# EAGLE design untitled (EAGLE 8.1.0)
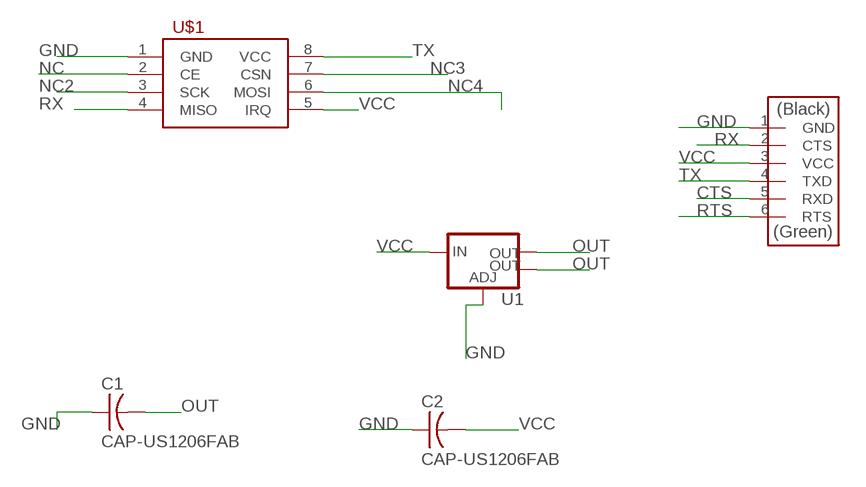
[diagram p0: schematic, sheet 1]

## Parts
C1  CAP-US1206FAB  [C1206FAB]
C2  CAP-US1206FAB  [C1206FAB]
U1  V_REG_LM1117SOT223  [SOT223]
U$1  NRF24L01+  [2X04_THRU]
U$2  FTDI-SMD-HEADER  [1X06SMD]

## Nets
CTS: U$2.5(RXD)
GND: C1.1 C2.1 U1.1(ADJ) U$1.1(GND) U$2.1(GND)
NC: U$1.2(CE)
NC2: U$1.3(SCK)
NC3: U$1.7(CSN)
NC4: U$1.6(MOSI)
OUT: C1.2 U1.2(OUT) U1.4(OUT)
RTS: U$2.6(RTS)
RX: U$1.4(MISO) U$2.2(CTS)
TX: U$1.8(VCC) U$2.4(TXD)
VCC: C2.2 U1.3(IN) U$1.5(IRQ) U$2.3(VCC)

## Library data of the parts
C1 C2 = fab:CAP-US
U1 = fab:V_REG_LM1117: Voltage Regulator LM1117 Standard adjustable voltage regulator but in SMD form. Spark Fun Electronics SKU : COM-00595; PROD_ID: VREG-08170
U$1 = fab:NRF24L01+: nRF24L01+ 2.4GHz Wireless Transceiver module
U$2 = fab:FTDI-SMD-HEADER

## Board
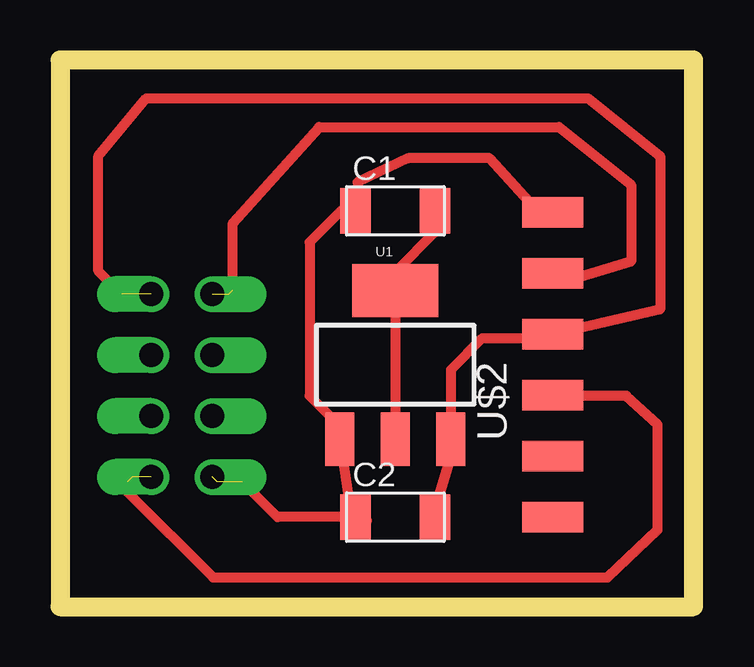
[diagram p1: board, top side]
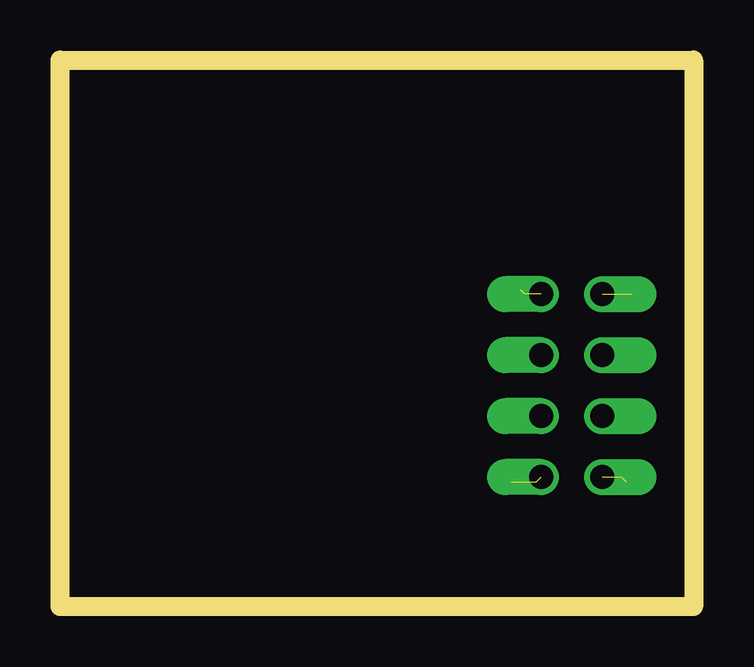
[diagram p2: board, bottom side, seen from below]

Size 26.4 x 22.8 mm. Coordinates in mm from the lower left corner, seen from the top.
Outline: 0,0 26.4,0 26.4,22.8 0,22.8 0,0
Copper layers (1*16): Top 0.035mm / dielectric 1.5mm / Bottom 0.035mm
Design rules "default": minimum track width 10mil, minimum drill 24mil, track to track 8mil, track to pad 8mil, pad to pad 8mil, via to via 8mil, smd to smd 8mil, copper to edge 40mil, drill to drill 8mil, minimum pad ring 10mil, minimum via ring 8mil, stop-mask expansion 4mil, vias tented up to drill 0mil, thermal gap 10mil

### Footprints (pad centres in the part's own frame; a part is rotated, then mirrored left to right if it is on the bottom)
C1206FAB = smd 1.27 x 1.905: 1 -1.651,0; 2 1.651,0
SOT223 = smd 1.219 x 2.235: 1 -2.311,-3.099; 2 0,-3.099; 3 2.311,-3.099 | smd 3.6 x 2.2: 4 0,3.099
2X04_THRU = drill 1 offset: 1 -1.27,3.81; 2 -1.27,1.27; 3 -1.27,-1.27; 4 -1.27,-3.81; 5 1.27,-3.81; 6 1.27,-1.27; 7 1.27,1.27; 8 1.27,3.81
1X06SMD = smd 2.54 x 1.27: 1 0,6.35; 2 0,3.81; 3 0,1.27; 4 0,-1.27; 5 0,-3.81; 6 0,-6.35

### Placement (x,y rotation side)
C1  13.97,16.51 0 top
C2  13.97,3.74 0 top
U1  13.97,10.09 0 top
U$1  5.08,9.22 180 top
U$2  20.53,10.09 0 top

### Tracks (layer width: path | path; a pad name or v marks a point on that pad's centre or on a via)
GND  (2 unrouted)
  Top 0.406: U$2.1 19.96,16.44 17.9,18.7 14.5,18.7 12.4,17.7 12.4,16.59 C1.1 11.71,16.51 10.4,15.2 10.4,8.8 11.6,7.6 11.6,7.05 U1.1 12.06,4.34 12.8,3.6 12.4,3.82 C2.1 9.06,3.74 7.6,5.2
OUT
  Top 0.406: C1.2 15.62,15.62 14,14 14,13.22 U1.4 U1.2
RX  (2 unrouted)
  Top 0.406: 7.2,13.2 7.2,16 10.8,20 20.8,20 23.8,17.6 23.8,14.4 21.2,13.6 20.83,13.6 U$2.2
TX  (2 unrouted)
  Top 0.406: 2.8,5.2 2.8,4.8 6.38,1.22 22.82,1.22 24.9,3.2 24.9,7.6 23.6,8.8 20.55,8.8 U$2.4
VCC  (1 unrouted)
  Top 0.406: C2.2 15.6,3.76 15.6,4 16.28,6.28 U1.3 16.28,9.88 17.6,11.2 20.37,11.2 U$2.3 20.77,11.6 21.6,11.6 25,12.4 25,18.8 22,21.2 3.6,21.2 1.6,18.8 1.6,14 2.57,13.03
(copper drawn outside any net)
  shapes: Bottom circle x17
